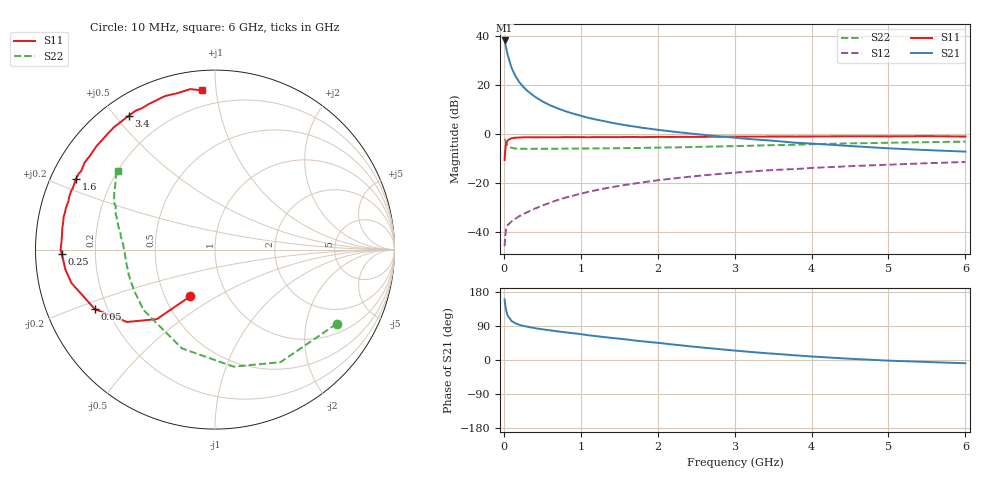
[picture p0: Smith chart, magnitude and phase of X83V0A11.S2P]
! SIEMENS Small Signal Semiconductors
! BFP136W
! Si NPN RF Bipolar Junction Transistor in SOT343
! VCE = 3 V  IC = 110 mA
! Common Emitter S-Parameters:  September  1994
# GHz  S  MA  R  50
!  f  S11  S21  S12  S22
! GHz  MAG  ANG  MAG  ANG  MAG  ANG  MAG  ANG
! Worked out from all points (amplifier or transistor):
!   40 points, 10 MHz to 6 GHz, reference 50 ohm
!   highest |S21| = 38.1 dB at 10 MHz (marker M1)
!   |S21| within 3 dB of that: start of sweep to 30.52 MHz
!   unconditionally stable (mu >= 1): 480.6 MHz to 2.904 GHz
!   at 200 MHz: K = 0.71, MSG = 27.3 dB, |S12| = -33.5 dB
!   at 1.5 GHz: K = 1.10, MAG = 10.7 dB, |S12| = -21.1 dB
!   at 6 GHz: K = 0.97, MSG = 2.1 dB, |S12| = -11.4 dB
!   S11 on the Smith chart (normalised r, x): 10 MHz: 0.67, -0.38; 50 MHz: 0.15, -0.23; 250 MHz: 0.08, -0.01; 1.6 GHz: 0.07, +0.24; 3.4 GHz: 0.08, +0.54; 6 GHz: 0.11, +0.92
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0.01  0.2947 -117.9  80.38 159.8  0.0052 69.9  0.7938 -31.4
0.02  0.5046 -129.9  68.49 143.0  0.0088 57.4  0.7256 -59.8
0.03  0.6354 -140.6  57.41 131.2  0.0115 48.8  0.6606 -80.9
0.05  0.7474 -153.7  40.7 117.3  0.0139 39.0  0.5806 -108.5
0.1  0.8211 -166.9  22.39 103.0  0.0166 37.6  0.5214 -139.7
0.15  0.8414 -172.5  15.21 96.8  0.0188 40.6  0.5057 -152.5
0.2  0.8465 -175.6  11.42 92.9  0.0212 43.3  0.5012 -159.4
0.25  0.8544 -178.4  9.214 90.1  0.0232 46.4  0.5007 -163.7
0.3  0.8602 -179.9  7.705 88.0  0.0254 48.8  0.4988 -166.7
0.4  0.8562 176.5  5.801 84.2  0.0301 53.6  0.4997 -170.7
0.5  0.8568 173.9  4.625 81.0  0.0348 56.3  0.5 -173.4
0.6  0.8591 172.0  3.855 78.4  0.0399 58.4  0.5009 -175.2
0.7  0.8594 169.6  3.322 75.5  0.0453 60.2  0.5022 -176.5
0.9  0.8612 166.1  2.603 70.6  0.0555 61.4  0.5045 -179.0
1.1  0.8599 161.7  2.133 65.2  0.0664 61.8  0.5078 179.3
1.6  0.8687 153.0  1.498 54.1  0.0929 60.1  0.5174 175.3
2.2  0.871 142.9  1.118 40.9  0.1241 55.6  0.5328 170.7
3.2  0.8842 125.9  0.789 21.4  0.1718 45.9  0.576 161.9
3.4  0.8871 122.9  0.749 18.1  0.181 43.8  0.5886 160.2
4.5  0.8997 108.0  0.57 3.3  0.2212 33.4  0.6451 150.5
5.5  0.9049 98.8  0.471 -5.2  0.2537 25.6  0.6838 143.9
6  0.8895 94.5  0.438 -8.6  0.2697 21.2  0.6984 141.0
